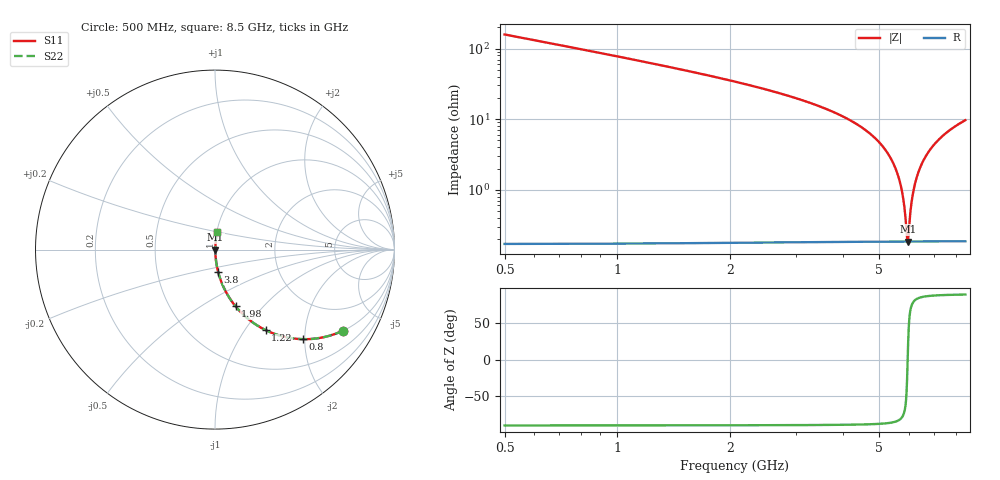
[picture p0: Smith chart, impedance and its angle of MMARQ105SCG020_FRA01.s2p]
! MMARQ105SCG020_FRA01  S-PARAMETER MODEL  ( General Type )
! Model Generated by TAIYO YUDEN Corporation (http://www.ty-top.com)
! Version 1.0
! TAIYO YUDEN Control No. 200326
! Copyright(c) 2020 TAIYO YUDEN CO.,LTD. All Rights Reserved.
! Product Description (link to TY-COMPAS)
! https://ds.yuden.co.jp/TYCOMPAS/or/detail?pn=MMARQ105SCG020BFRA01&u=M
! Products Name : Multilayer Ceramic Capacitors
! Characteristics :
!  Capacitance : 2 pF , Rated Voltage : 250V , TCC : CG / C0G
!  Case Size : 1.0 x 0.5 / 0.039 x 0.02 [mm/inch] , Thickness : 0.5 / 0.02 [mm/inch]
!  (Conditions: Temperature = 25 degC , DC Bias Current/Voltage = 0A / 0V)
! External Node Assignments :
!  1  o---| |---o  2
! GND o---------o GND
! Frequency Range : 500MHz  -  8.5GHz  [ 401 STEP ]
# MHz S RI R 50
! Freq[MHz].  S11 Real  S11 Imag  S21 Real  S21 Imag  S12 Real  S12 Imag  S22 Real  S22 Imag
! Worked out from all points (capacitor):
!   401 points, 500 MHz to 8.5 GHz, reference 50 ohm
!   read as one part in series: C = 2 pF near 540 MHz
!   lowest |Z| = 185 mohm at 5.96 GHz (marker M1)
!   series resonance near 5.96 GHz, so ESL is about 360 pH
!   S11 on the Smith chart (normalised r, x): 500 MHz: 1.00, -3.17; 800 MHz: 1.00, -1.96; 1.22 GHz: 1.00, -1.25; 1.98 GHz: 1.00, -0.72; 3.8 GHz: 1.00, -0.25; 8.5 GHz: 1.00, +0.19
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500  0.7145 -0.4511  0.2855 0.4511  0.2855 0.4511  0.7145 -0.4511
800  0.4891 -0.499  0.5109 0.499  0.5109 0.499  0.4891 -0.499
1220  0.282 -0.4486  0.718 0.4486  0.718 0.4486  0.282 -0.4486
1840  0.1342 -0.3387  0.8658 0.3387  0.8658 0.3387  0.1342 -0.3387
1980  0.1149 -0.3164  0.8851 0.3164  0.8851 0.3164  0.1149 -0.3164
3180  0.0328 -0.1731  0.9672 0.1731  0.9672 0.1731  0.0328 -0.1731
3800  0.017 -0.1221  0.983 0.1221  0.983 0.1221  0.017 -0.1221
4500  0.00757 -0.0754  0.9924 0.0754  0.9924 0.0754  0.00757 -0.0754
5040  0.00386 -0.0448  0.9961 0.0448  0.9961 0.0448  0.00386 -0.0448
5420  0.00249 -0.0253  0.9975 0.0253  0.9975 0.0253  0.00249 -0.0253
5680  0.00201 -0.0128  0.998 0.0128  0.998 0.0128  0.00201 -0.0128
5760  0.00193 -0.00911  0.9981 0.00911  0.9981 0.00911  0.00193 -0.00911
5840  0.00188 -0.00543  0.9981 0.00543  0.9981 0.00543  0.00188 -0.00543
5920  0.00185 -0.00181  0.9981 0.00181  0.9981 0.00181  0.00185 -0.00181
5960  0.00185 -1.16e-05  0.9981 1.16e-05  0.9981 1.16e-05  0.00185 -1.16e-05
6000  0.00185 0.00177  0.9981 -0.00177  0.9981 -0.00177  0.00185 0.00177
6080  0.00188 0.0053  0.9981 -0.0053  0.9981 -0.0053  0.00188 0.0053
6140  0.00192 0.00792  0.9981 -0.00792  0.9981 -0.00792  0.00192 0.00792
6340  0.00213 0.0165  0.9979 -0.0165  0.9979 -0.0165  0.00213 0.0165
6680  0.00278 0.0304  0.9972 -0.0304  0.9972 -0.0304  0.00278 0.0304
7180  0.00435 0.0498  0.9957 -0.0498  0.9957 -0.0498  0.00435 0.0498
8500  0.0111 0.0957  0.9889 -0.0957  0.9889 -0.0957  0.0111 0.0957
